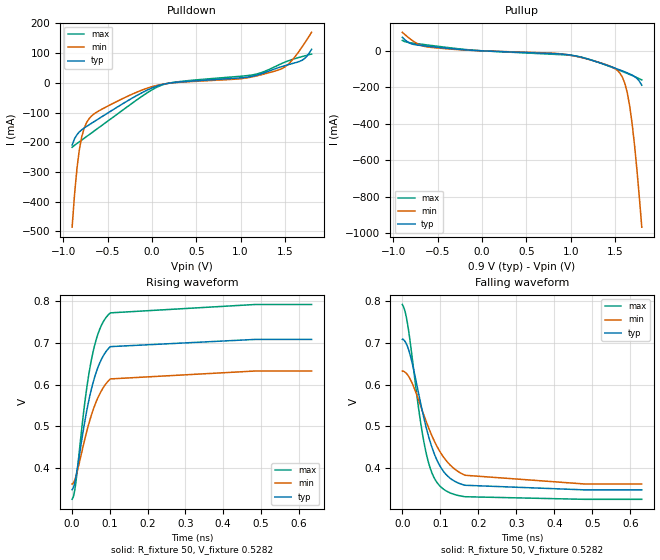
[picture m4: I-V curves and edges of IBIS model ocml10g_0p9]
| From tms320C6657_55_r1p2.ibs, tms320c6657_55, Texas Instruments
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|   Model Cell OCML10G_0P9
|OCML10G_0P9
[Model]   ocml10g_0p9
Model_type   Output
Polarity   Non-Inverting
Cref =  1PF
Rref =  1M
Vref =  0V
Vmeas =  0.5282V
C_comp   1p   1p   1p
| Input capacitance of this buffer has no significance since this is output
|only buffer
[Temperature Range]   25   125   -40
[Voltage Range]   0.9   0.81   0.99
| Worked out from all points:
|   slope of the pulldown table from 0 to 0.135 V, typ, clamps not added: 10.4 ohm
|   slope of the pullup table from 0 to 0.135 V, typ, clamps not added: 49.9 ohm
|   rising waveform, R_fixture 50, V_fixture 0.5282: 20-80 % time 48.9ps typ, 53.6ps min, 44.4ps max; typ from 0.348 V to 0.708 V
|   falling waveform, R_fixture 50, V_fixture 0.5282: 20-80 % time 61ps typ, 80.4ps min, 46.2ps max; typ from 0.708 V to 0.348 V
[Pulldown]
|   voltage   I(typ)   I(min)   I(max)
-900mV    -209.1mA   -485.6mA   -216.9mA
-872.7mV  -188.1mA   -375.5mA   -210.2mA
-845.5mV  -174.4mA   -288.2mA   -204.2mA
-790.9mV  -158mA     -180.6mA   -192.4mA
-736.4mV  -146.7mA   -133.3mA   -180.6mA
-654.5mV  -131mA     -105mA     -162.8mA
109.1mV   -6.262mA   -5.289mA   -8.037mA
1.145V    22.85mA    20.87mA    27.34mA
1.445V    52.86mA    45.26mA    62.5mA
1.555V    62.5mA     67.58mA    75.72mA
1.691V    75.57mA    120mA      88.08mA
1.8V      112.8mA    169.9mA    96.75mA
[Pullup]
|   voltage   I(typ)   I(min)   I(max)
-900mV    74.46mA    101.6mA    56.94mA
-790.9mV  37.57mA    58.12mA    43.22mA
-627.3mV  25.92mA    22.39mA    32.93mA
900mV     -17.74mA   -17.13mA   -21.18mA
1.145V    -38.5mA    -39.88mA   -37.93mA
1.527V    -99.99mA   -107.9mA   -102.3mA
1.609V    -115.3mA   -178.6mA   -118.4mA
1.664V    -126.4mA   -302.1mA   -129.4mA
1.691V    -132.6mA   -398.2mA   -135.1mA
1.718V    -140.3mA   -516.1mA   -141mA
1.745V    -150.7mA   -652.5mA   -146.9mA
1.8V      -188.7mA   -966.3mA   -159.3mA
[Ramp]
| variable   typ   min   max
dV/dt_f   0.217884/61.265159p   0.163398/80.698965p   0.281988/46.34576p
dV/dt_r   0.217176/49.539846p   0.16524/55.43001p   0.279924/44.503009p
R_load = 50
[Rising Waveform]
R_fixture = 50
V_fixture = 0.5282
V_fixture_min = 0.4972
V_fixture_max = 0.5585
|   time   V(typ)   V(min)   V(max)
0s        348.4mV    362.1mV    325.5mV
5.271ps   359.1mV    367.8mV    339mV
9.271ps   375.6mV    378mV      361.5mV
35.27ps   520.2mV    475.4mV    568.6mV
43.27ps   557.8mV    503mV      618.8mV
53.27ps   596.9mV    533mV      668.7mV
63.27ps   627.9mV    557.8mV    705.9mV
75.27ps   655.9mV    581.3mV    737mV
101.3ps   690.7mV    613.5mV    771.5mV
634.7ps   707.9mV    632.4mV    791.5mV
[Falling Waveform]
R_fixture = 50
V_fixture = 0.5282
V_fixture_min = 0.4972
V_fixture_max = 0.5585
|   time   V(typ)   V(min)   V(max)
0s        708.2mV    632.4mV    792mV
6.977ps   703.7mV    629.9mV    775.9mV
14.98ps   687.9mV    621.9mV    738.8mV
44.98ps   569.5mV    557.5mV    529.4mV
60.98ps   504.1mV    516.2mV    443.4mV
78.98ps   446.9mV    475.1mV    386mV
105ps     396.3mV    430.8mV    351.8mV
131ps     372mV      402.7mV    338.5mV
165ps     358.6mV    382.6mV    331.1mV
630.4ps   347.5mV    361.6mV    324.9mV
